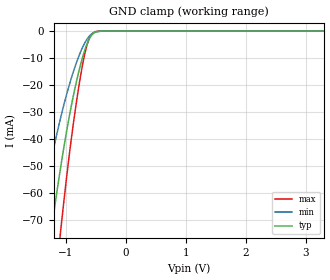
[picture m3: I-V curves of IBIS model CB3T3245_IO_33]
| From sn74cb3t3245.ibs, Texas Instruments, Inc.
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[Model]   CB3T3245_IO_33
Model_type  Terminator
| variable   typ   min   max
C_comp   3.94pF   3.22pF   4.29pF
| C_tri-state   3.94pF   3.22pF   4.29pF
[Temperature Range]   40   100   -40
| Ambient temperature   25   85   -40
[Voltage range]   3.3   3   3.6
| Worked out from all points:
|   GND clamp passes 1 mA (typ) near -0.54 V on its own axis
[GND Clamp]
| CB3T3245_IO_33
|   Voltage   I(typ)   I(min)   I(max)
-5V       -923.7mA   -700.9mA   -1.157A
-1.505V   -119.4mA   -78.18mA   -171.9mA
-1.455V   -110.3mA   -71.95mA   -159.4mA
-1.24V    -73.63mA   -47.28mA   -107.8mA
-1.095V   -51.65mA   -32.87mA   -75.81mA
-1.075V   -48.84mA   -31.04mA   -71.64mA
-920mV    -29.01mA   -18.28mA   -41.92mA
-765mV    -13.36mA   -8.294mA   -18.03mA
-655mV    -5.244mA   -3.27mA    -5.793mA
-595mV    -2.383mA   -1.563mA   -2.065mA
-540mV    -897uA     -662.9uA   -562.3uA
3.3V      299pA      11.27nA    65.82pA
